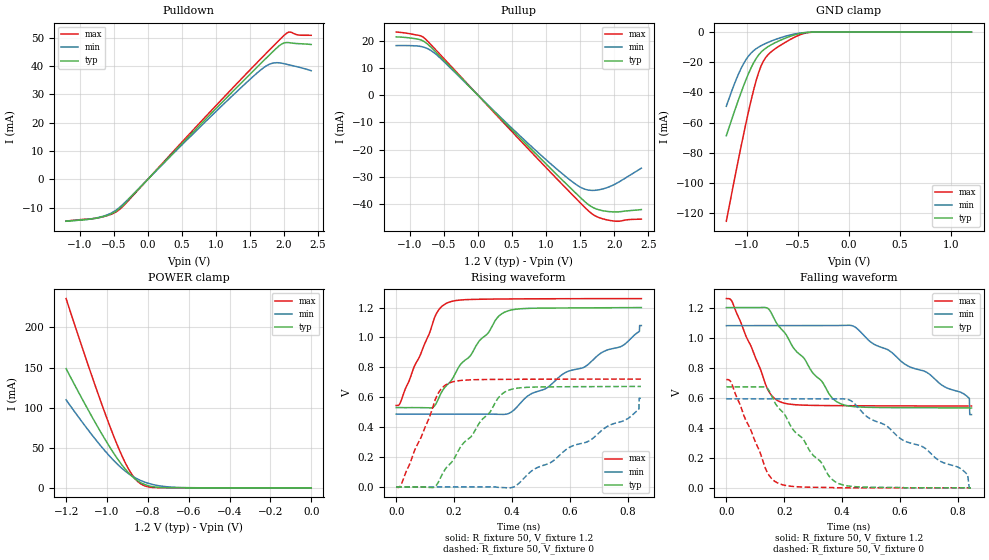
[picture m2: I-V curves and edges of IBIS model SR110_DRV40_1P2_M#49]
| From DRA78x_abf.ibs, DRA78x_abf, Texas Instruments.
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| Model based on original model for DDR_SEIOPB_V
|   Sub model SR110_DRV40_1P2
[model]   SR110_DRV40_1P2_M#49
|[Description]  [1.2V-I/O-X-X]
|   , ,
|[Input Load]
|[Output Drive]
|Voltage   1.2V
|Mode   I/O
Model_type   I/O
Polarity   Non-Inverting
Enable   Active-Low
Vinl =  0.47
Vinh =  0.73
Cref =  15.0000pF
Rref =  100.0000M
Vref =  0V
Vmeas =  0.6
C_comp   2p   2p   2p
[Model Spec]
Vinl   0.47   0.41   0.50
Vinh   0.73   0.67   0.76
[Receiver Thresholds]
Tslew_ac = 5n
Vth = 0.6
Vth_max = 0.63
Vth_min = 0.54
Vinh_ac = 0.22
Vinh_dc = 0.13
Vinl_ac = -0.22
Vinl_dc = -0.13
[Temperature Range]   25   125   -40
[Voltage Range]   1.2   1.08   1.26
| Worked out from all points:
|   slope of the pulldown table from 0 to 0.18 V, typ, clamps not added: 39.6 ohm
|   slope of the pullup table from 0 to 0.18 V, typ, clamps not added: 39.1 ohm
|   GND clamp passes 1 mA (typ) near -0.48 V on its own axis
|   POWER clamp passes 1 mA (typ) near -0.76 V on its own axis
|   rising waveform, R_fixture 50, V_fixture 1.2: 20-80 % time 162ps typ, 341ps min, 89.9ps max; typ from 0.531 V to 1.2 V
|   rising waveform, R_fixture 50, V_fixture 0: 20-80 % time 159ps typ, 335ps min, 88.9ps max; typ from 0 V to 0.672 V
|   falling waveform, R_fixture 50, V_fixture 1.2: 20-80 % time 158ps typ, 328ps min, 89ps max; typ from 1.2 V to 0.531 V
|   falling waveform, R_fixture 50, V_fixture 0: 20-80 % time 160ps typ, 331ps min, 89.8ps max; typ from 0.672 V to 0 V
[POWER_clamp]
-1.2V     148.6mA    109.7mA    235.9mA
-1.115V   108mA      79.97mA    170.5mA
-1.055V   80.16mA    59.93mA    125.3mA
-1.006V   59.04mA    45.03mA    90.73mA
-957.6mV  39.59mA    31.69mA    58.49mA
-921.2mV  26.75mA    23.11mA    36.96mA
-897mV    19.41mA    18.26mA    24.7mA
-860.6mV  10.74mA    12.35mA    10.83mA
-836.4mV  6.696mA    9.316mA    5.268mA
-787.9mV  2.052mA    4.939mA    818.3uA
-666.7mV  49.08uA    692.2uA    5.202uA
0V        48.89nA    205.6nA    269.9nA
[Pulldown]
-1.2V     -14.8mA    -14.74mA   -14.71mA
-690.9mV  -13.39mA   -13.26mA   -13.4mA
-509.1mV  -11.88mA   -11.54mA   -12.04mA
-400mV    -9.96mA    -9.599mA   -10.33mA
1.018V    25.39mA    24.35mA    26.45mA
1.527V    37.74mA    35.87mA    39.28mA
1.745V    42.94mA    40.13mA    44.66mA
1.855V    45.5mA     41.09mA    47.32mA
1.964V    47.72mA    41.01mA    49.95mA
2.073V    48.25mA    40.41mA    51.99mA
2.218V    47.89mA    39.59mA    50.92mA
2.4V      47.6mA     38.35mA    50.84mA
[Pullup]
-1.2V     21.34mA    18.16mA    23.12mA
-836.4mV  20.22mA    17.83mA    21.7mA
-763.6mV  19.2mA     17.3mA     20.39mA
-654.5mV  16.69mA    15.75mA    17.55mA
836.4mV   -21.16mA   -19.98mA   -22.26mA
1.273V    -31.93mA   -29.49mA   -33.59mA
1.527V    -38.06mA   -34.03mA   -40.07mA
1.6V      -39.68mA   -34.68mA   -41.87mA
1.709V    -41.42mA   -34.9mA    -44.05mA
1.855V    -42.44mA   -34.22mA   -45.47mA
2.036V    -42.8mA    -32.31mA   -46.22mA
2.4V      -41.95mA   -26.76mA   -45.45mA
[GND_clamp]
-1.2V     -68.74mA   -49.24mA   -125.5mA
-1.127V   -53.92mA   -35.5mA    -100.1mA
-1.055V   -39.92mA   -23.99mA   -75.5mA
-981.8mV  -27.37mA   -15.83mA   -52.4mA
-909.1mV  -17.63mA   -11.09mA   -32.41mA
-860.6mV  -13.38mA   -9.079mA   -22.59mA
-836.4mV  -11.86mA   -8.241mA   -19.18mA
-787.9mV  -9.515mA   -6.746mA   -14.76mA
-739.4mV  -7.652mA   -5.419mA   -11.95mA
-521.2mV  -1.657mA   -1.168mA   -3.09mA
-375.8mV  -108.2uA   -128.9uA   -198.1uA
1.2V      48.89nA    308.5nA    224.4nA
[Ramp]
dV/dt_f 0.40220104/0.15836549n 0.35721706/0.32913171n 0.42977113/89.184827p
dV/dt_r 0.40622367/0.16069349n 0.35925006/0.3384103n 0.43555875/89.63621p
R_load = 50
[Rising Waveform]
R_fixture = 50
V_fixture = 1.2
V_fixture_min = 1.08
V_fixture_max = 1.26
0s        531.3mV    487.5mV    545.3mV
13.5ps    531.2mV    487.5mV    560.6mV
125.8ps   531.6mV    487.5mV    1.095V
145.8ps   589.3mV    487.4mV    1.182V
176.7ps   684.6mV    487.5mV    1.232V
347ps     1.127V     485.5mV    1.257V
384.8ps   1.177V     489mV      1.258V
581.9ps   1.198V     762.4mV    1.259V
786.9ps   1.199V     950.8mV    1.26V
847.1ps   1.2V       1.08V      1.26V
[Rising Waveform]
R_fixture = 50
V_fixture = 0
V_fixture_min = 0
V_fixture_max = 0
0s        0V         0V         0V
19ps      0V         0V         23.69mV
129.8ps   -2.951mV   0V         556.1mV
179.3ps   141.9mV    0V         692.4mV
387.2ps   646.4mV    -5.98mV    720.1mV
596.8ps   670.5mV    262.7mV    721.3mV
801.5ps   671.6mV    458.6mV    721.6mV
838.8ps   671.7mV    521.7mV    721.6mV
839.3ps   672.4mV    592.8mV    721.6mV
845.3ps   672.4mV    592.8mV    721.6mV
[Falling Waveform]
R_fixture = 50
V_fixture = 1.2
V_fixture_min = 1.08
V_fixture_max = 1.26
0s        1.2V       1.08V      1.26V
20.8ps    1.2V       1.08V      1.237V
139.4ps   1.199V     1.08V      670.2mV
181.6ps   1.075V     1.08V      576.3mV
394.1ps   560.3mV    1.081V     547mV
440.7ps   540.7mV    1.075V     546.4mV
821.1ps   532.2mV    625mV      545mV
839.8ps   532.1mV    595.1mV    545mV
841.1ps   531.3mV    487.5mV    544.9mV
847.1ps   531.3mV    487.5mV    544.9mV
[Falling Waveform]
R_fixture = 50
V_fixture = 0
V_fixture_min = 0
V_fixture_max = 0
0s        672.4mV    592.8mV    721mV
18.8ps    672.4mV    592.8mV    693mV
135.9ps   669.6mV    592.8mV    125.6mV
179.4ps   534.8mV    592.8mV    30.24mV
357.5ps   71.76mV    592.7mV    2.194mV
390.4ps   26.65mV    593.1mV    0V
807.1ps   0V         131mV      0V
834ps     0V         86.6mV     0V
839.3ps   0V         0V         0V
845.3ps   0V         0V         0V
